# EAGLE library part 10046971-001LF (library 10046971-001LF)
Standard Card Edge Connectors 2.54MM VERT RECPT 2 ROW 64 CON Source: Datasheet
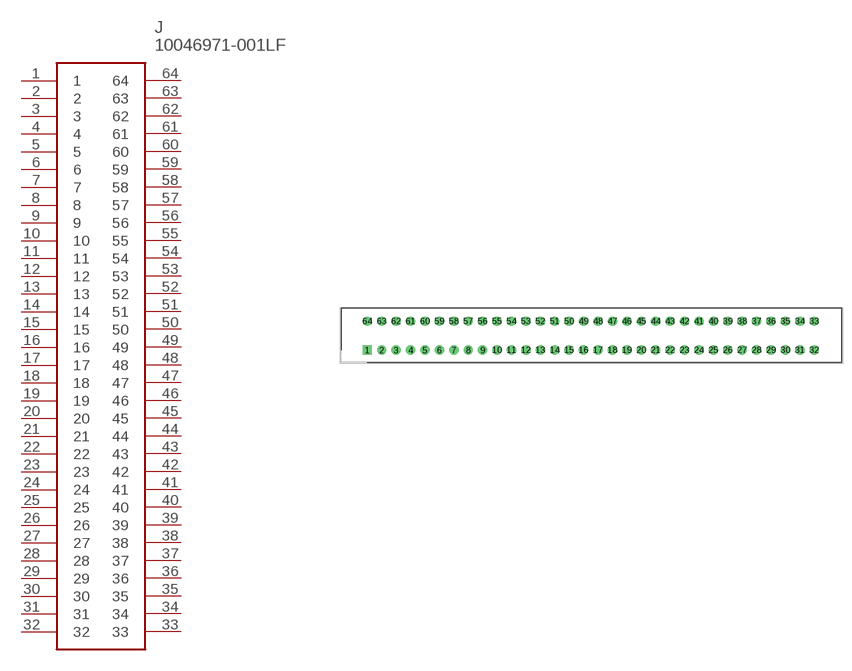
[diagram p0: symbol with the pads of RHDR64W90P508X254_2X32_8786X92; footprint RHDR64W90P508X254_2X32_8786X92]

Designator prefix J

## 10046971-001LF (Arrow_Part_Number: 10046971-001LF; Arrow_Price-Stock: https://www.arrow.com/en/products/10046971-001lf/amphenol-fci?region=nac; Description: Standard Card Edge Connectors 2.54MM VERT RECPT 2 ROW 64 CON; Height: 15.49mm; Manufacturer_Name: Amphenol; Manufacturer_Part_Number: 10046971-001LF; Mouser_Part_Number: 649-10046971-001LF; Mouser_Price-Stock: https://www.mouser.co.uk/ProductDetail/Amphenol-FCI/10046971-001LF?qs=U4pz39agNJCIvqufzwZVMg%3D%3D)  [RHDR64W90P508X254_2X32_8786X92]
1  1
2  2
3  3
4  4
5  5
6  6
7  7
8  8
9  9
10  10
11  11
12  12
13  13
14  14
15  15
16  16
17  17
18  18
19  19
20  20
21  21
22  22
23  23
24  24
25  25
26  26
27  27
28  28
29  29
30  30
31  31
32  32
33  33
34  34
35  35
36  36
37  37
38  38
39  39
40  40
41  41
42  42
43  43
44  44
45  45
46  46
47  47
48  48
49  49
50  50
51  51
52  52
53  53
54  54
55  55
56  56
57  57
58  58
59  59
60  60
61  61
62  62
63  63
64  64

## Footprint RHDR64W90P508X254_2X32_8786X92 (pad centres in mm)
10046971-001LF
drill 1.1 pad 1.65 square: 1 0,0
drill 1.1 pad 1.65: 2 2.54,0; 3 5.08,0; 4 7.62,0; 5 10.16,0; 6 12.7,0; 7 15.24,0; 8 17.78,0; 9 20.32,0; 10 22.86,0; 11 25.4,0; 12 27.94,0; 13 30.48,0; 14 33.02,0; 15 35.56,0; 16 38.1,0; 17 40.64,0; 18 43.18,0; 19 45.72,0; 20 48.26,0; 21 50.8,0; 22 53.34,0; 23 55.88,0; 24 58.42,0; 25 60.96,0; 26 63.5,0; 27 66.04,0; 28 68.58,0; 29 71.12,0; 30 73.66,0; 31 76.2,0; 32 78.74,0; 33 78.74,5.08; 34 76.2,5.08; 35 73.66,5.08; 36 71.12,5.08; 37 68.58,5.08; 38 66.04,5.08; 39 63.5,5.08; 40 60.96,5.08; 41 58.42,5.08; 42 55.88,5.08; 43 53.34,5.08; 44 50.8,5.08; 45 48.26,5.08; 46 45.72,5.08; 47 43.18,5.08; 48 40.64,5.08; 49 38.1,5.08; 50 35.56,5.08; 51 33.02,5.08; 52 30.48,5.08; 53 27.94,5.08; 54 25.4,5.08; 55 22.86,5.08; 56 20.32,5.08; 57 17.78,5.08; 58 15.24,5.08; 59 12.7,5.08; 60 10.16,5.08; 61 7.62,5.08; 62 5.08,5.08; 63 2.54,5.08; 64 0,5.08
